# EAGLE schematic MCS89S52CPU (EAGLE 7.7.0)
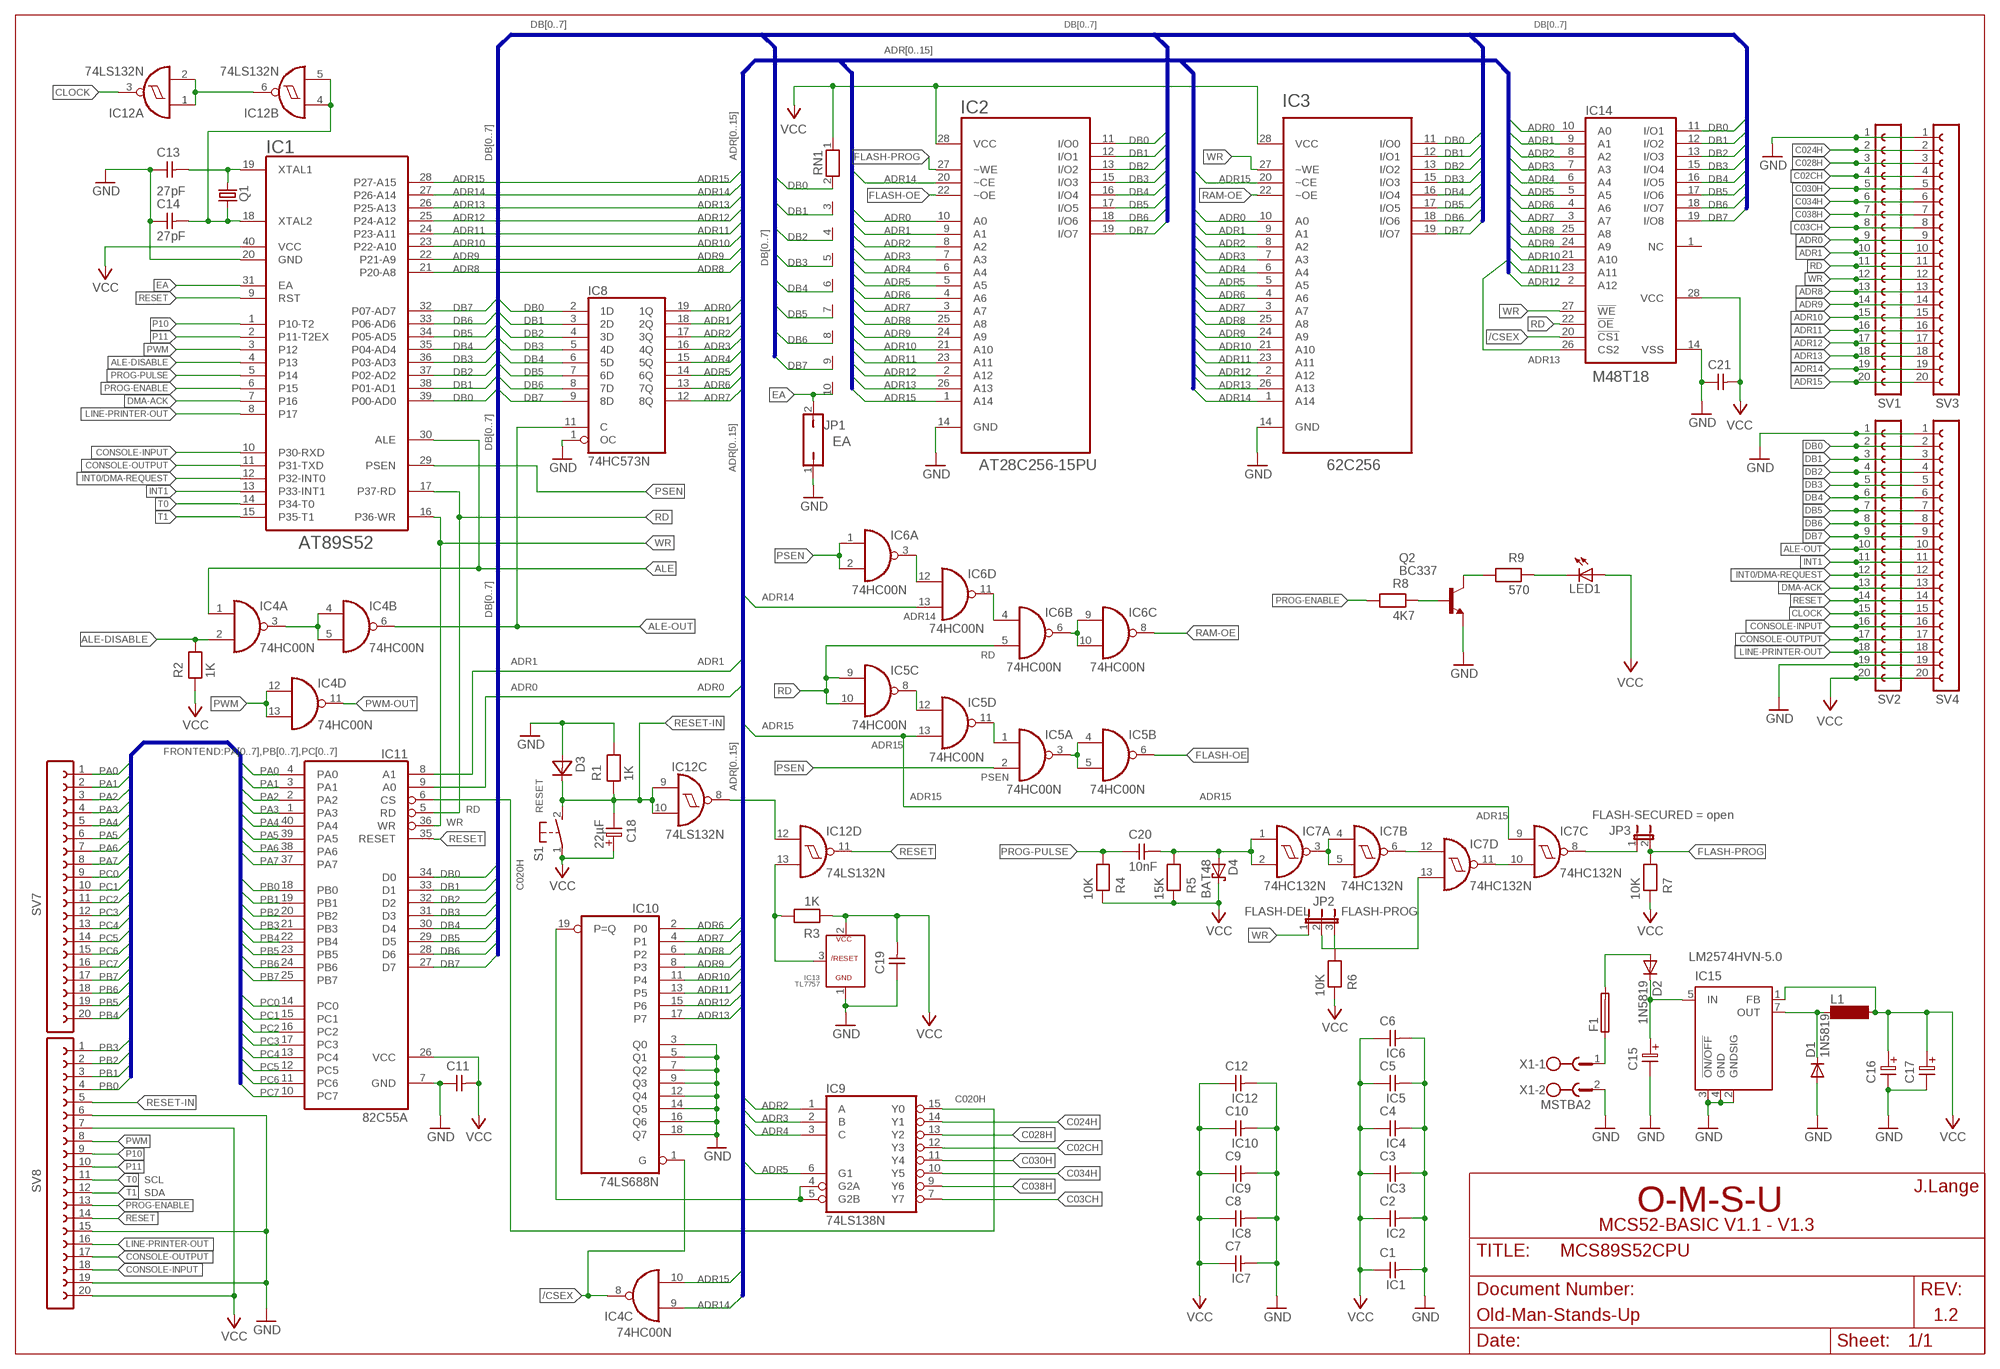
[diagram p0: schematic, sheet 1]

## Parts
C1  CAPNP-5  [C-5]
C2  CAPNP-5  [C-5]
C3  CAPNP-5  [C-5]
C4  CAPNP-5  [C-5]
C5  CAPNP-5  [C-5]
C6  CAPNP-5  [C-5]
C7  CAPNP-5  [C-5]
C8  CAPNP-5  [C-5]
C9  CAPNP-5  [C-5]
C10  CAPNP-5  [C-5]
C11  CAPNP-5  [C-5]
C12  CAPNP-5  [C-5]
C13  27pF  CAPNP-2,5  [C-2,5]
C14  27pF  CAPNP-2,5  [C-2,5]
C15  ELC-5  [ES-5]
C16  ELC-5  [ES-5]
C17  ELC-5  [ES-5]
C18  22µF  ELC-2,5  [ES-2,5]
C19  CAPNP-5  [C-5]
C20  10nF  CAPNP-5  [C-5]
C21  CAPNP-5  [C-5]
D1  1N5819  DIODE-DO41-7.6  [DO41-7.6]
D2  1N5819  DIODE-DO41-7.6  [DO41-7.6]
D3  DIODE-7,5  [D-7,5]
D4  BAT48  BAT42  [DO35-10]
F1  TR5  [TR5]
IC1  AT89S52  8052N  [DIL40]
IC2  AT28C256-15PU  [DIP254P1524X482-28]
IC3  62C256  AT28C256-15PU  [DIP254P1524X482-28]
IC4  74HC00N  [DIL14]
IC5  74HC00N  [DIL14]
IC6  74HC00N  [DIL14]
IC7  74HC132N  [DIL14]
IC8  74HC573N  [DIL20]
IC9  74LS138N  [DIL16]
IC10  74LS688N  [DIL20]
IC11  82C55A  [DIL40]
IC12  74LS132N  [DIL14]
IC13  TL7757  [TO92]
IC14  M48T18  6264A  [DIL28-6]
IC15  LM2574HVN-5.0  [DIL08]
JP1  JP1Q  [JP1]
JP2  JP2E  [JP2]
JP3  JP1E  [JP1]
L1  12K100-7,5  [12K100-7.5]
LED1  LED5MM  [LED5MM]
Q1  CRYSTALHC49S  [HC49/S]
Q2  BC337  [TO92]
R1  1K  RESEU-7,5  [R-7,5]
R2  1K  RESEU-7,5  [R-7,5]
R3  1K  RESEU-7,5  [R-7,5]
R4  10K  RESEU-7,5  [R-7,5]
R5  15K  RESEU-7,5  [R-7,5]
R6  10K  RESEU-7,5  [R-7,5]
R7  10K  RESEU-7,5  [R-7,5]
R8  4K7  RESEU-7,5  [R-7,5]
R9  570  RESEU-7,5  [R-7,5]
RN1  RN09  [RN-10]
S1  31-XX  [B3F-31XX]
SV1  FE20W  [FE20W]
SV2  FE20W  [FE20W]
SV3  FE20-1  [FE20]
SV4  FE20-1  [FE20]
SV7  FE20-1  [FE20]
SV8  FE20-1  [FE20]
X1  MSTBA2  [MSTBA2]

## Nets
/CSEX: IC4.8(C:O) IC10.1(G) IC14.20(!CS1)
ADR0: IC2.10(A0) IC3.10(A0) IC8.19(1Q) IC11.9(A0) IC14.10(A0) SV1.9 SV3.9
ADR1: IC2.9(A1) IC3.9(A1) IC8.18(2Q) IC11.8(A1) IC14.9(A1) SV1.10 SV3.10
ADR2: IC2.8(A2) IC3.8(A2) IC8.17(3Q) IC9.1(A) IC14.8(A2)
ADR3: IC2.7(A3) IC3.7(A3) IC8.16(4Q) IC9.2(B) IC14.7(A3)
ADR4: IC2.6(A4) IC3.6(A4) IC8.15(5Q) IC9.3(C) IC14.6(A4)
ADR5: IC2.5(A5) IC3.5(A5) IC8.14(6Q) IC9.6(G1) IC14.5(A5)
ADR6: IC2.4(A6) IC3.4(A6) IC8.13(7Q) IC10.2(P0) IC14.4(A6)
ADR7: IC2.3(A7) IC3.3(A7) IC8.12(8Q) IC10.4(P1) IC14.3(A7)
ADR8: IC1.21(P20-A8) IC2.25(A8) IC3.25(A8) IC10.6(P2) IC14.25(A8) SV1.13 SV3.13
ADR9: IC1.22(P21-A9) IC2.24(A9) IC3.24(A9) IC10.8(P3) IC14.24(A9) SV1.14 SV3.14
ADR10: IC1.23(P22-A10) IC2.21(A10) IC3.21(A10) IC10.11(P4) IC14.21(A10) SV1.15 SV3.15
ADR11: IC1.24(P23-A11) IC2.23(A11) IC3.23(A11) IC10.13(P5) IC14.23(A11) SV1.16 SV3.16
ADR12: IC1.25(P24-A12) IC2.2(A12) IC3.2(A12) IC10.15(P6) IC14.2(A12) SV1.17 SV3.17
ADR13: IC1.26(P25-A13) IC2.26(A13) IC3.26(A13) IC10.17(P7) IC14.26(CS2) SV1.18 SV3.18
ADR14: IC1.27(P26-A14) IC2.20(~CE) IC3.1(A14) IC4.9(C:I0) IC6.13(D:I1) SV1.19 SV3.19
ADR15: IC1.28(P27-A15) IC2.1(A14) IC3.20(~CE) IC4.10(C:I1) IC5.13(D:I1) IC7.9(C:I0) SV1.20 SV3.20
ALE: IC1.30(ALE) IC4.1(A:I0)
ALE-DISABLE: IC1.4(P13) IC4.2(A:I1) R2.2
ALE-OUT: IC4.6(B:O) IC8.11(C) SV2.10 SV4.10
C02CH: IC9.12(Y3) SV1.4 SV3.4
C03CH: IC9.7(Y7) SV1.8 SV3.8
C020H: IC9.15(Y0) IC11.6(CS)
C024H: IC9.14(Y1) SV1.2 SV3.2
C028H: IC9.13(Y2) SV1.3 SV3.3
C030H: IC9.11(Y4) SV1.5 SV3.5
C034H: IC9.10(Y5) SV1.6 SV3.6
C038H: IC9.9(Y6) SV1.7 SV3.7
CLOCK: IC12.3(A:O) SV2.15 SV4.15
CONSOLE-INPUT: IC1.10(P30-RXD) SV2.16 SV4.16 SV8.18
CONSOLE-OUTPUT: IC1.11(P31-TXD) SV2.17 SV4.17 SV8.17
DB0: IC1.39(P00-AD0) IC2.11(I/O0) IC3.11(I/O0) IC8.2(1D) IC11.34(D0) IC14.11(I/O1) RN1.2 SV2.2 SV4.2
DB1: IC1.38(P01-AD1) IC2.12(I/O1) IC3.12(I/O1) IC8.3(2D) IC11.33(D1) IC14.12(I/O2) RN1.3 SV2.3 SV4.3
DB2: IC1.37(P02-AD2) IC2.13(I/O2) IC3.13(I/O2) IC8.4(3D) IC11.32(D2) IC14.13(I/O3) RN1.4 SV2.4 SV4.4
DB3: IC1.36(P03-AD3) IC2.15(I/O3) IC3.15(I/O3) IC8.5(4D) IC11.31(D3) IC14.15(I/O4) RN1.5 SV2.5 SV4.5
DB4: IC1.35(P04-AD4) IC2.16(I/O4) IC3.16(I/O4) IC8.6(5D) IC11.30(D4) IC14.16(I/O5) RN1.6 SV2.6 SV4.6
DB5: IC1.34(P05-AD5) IC2.17(I/O5) IC3.17(I/O5) IC8.7(6D) IC11.29(D5) IC14.17(I/O6) RN1.7 SV2.7 SV4.7
DB6: IC1.33(P06-AD6) IC2.18(I/O6) IC3.18(I/O6) IC8.8(7D) IC11.28(D6) IC14.18(I/O7) RN1.8 SV2.8 SV4.8
DB7: IC1.32(P07-AD7) IC2.19(I/O7) IC3.19(I/O7) IC8.9(8D) IC11.27(D7) IC14.19(I/O8) RN1.9 SV2.9 SV4.9
DMA-ACK: IC1.7(P16) SV2.13 SV4.13
EA: IC1.31(EA) JP1.2 RN1.10
FLASH-OE: IC2.22(~OE) IC5.6(B:O)
FLASH-PROG: IC2.27(~WE) JP3.2 R7.1
GND: C1.2 C2.2 C3.2 C4.2 C5.2 C6.2 C7.2 C8.2 C9.2 C10.2 C11.1 C12.2 C13.1 C14.1 C15.2 C16.2 C17.2 C19.1 C21.1 D1.A D3.1(A) IC1.20(GND) IC2.14(GND) IC3.14(GND) IC8.1(OC) IC10.3(Q0) IC10.5(Q1) IC10.7(Q2) IC10.9(Q3) IC10.12(Q4) IC10.14(Q5) IC10.16(Q6) IC10.18(Q7) IC11.7(GND) IC13.1(GND) IC14.14(VSS) IC15.2(GNDSIG) IC15.3(!ON/OFF) IC15.4(GND) JP1.1 Q2.1(E) R1.2 SV1.1 SV2.1 SV2.19 SV3.1 SV4.1 SV4.19 SV8.6 SV8.15 SV8.19 X1.2
INT0/DMA-REQUEST: IC1.12(P32-INT0) SV2.12 SV4.12
INT1: IC1.13(P33-INT1) SV2.11 SV4.11
LINE-PRINTER-OUT: IC1.8(P17) SV2.18 SV4.18 SV8.16
N$1: D1.C IC15.7(OUT) L1.1
N$2: C13.2 IC1.19(XTAL1) Q1.2
N$3: C15.1 D2.C IC15.5(IN)
N$4: F1.1 X1.1
N$5: D2.A F1.2
N$6: C14.2 IC1.18(XTAL2) IC12.4(B:I0) IC12.5(B:I1) Q1.1
N$7: IC12.13(D:I1) IC13.3(/RESET) R3.2
N$8: IC4.3(A:O) IC4.4(B:I0) IC4.5(B:I1)
N$9: IC12.1(A:I0) IC12.2(A:I1) IC12.6(B:O)
N$10: IC5.8(C:O) IC5.12(D:I0)
N$11: IC5.1(A:I0) IC5.11(D:O)
N$12: IC12.8(C:O) IC12.12(D:I0)
N$13: IC5.3(A:O) IC5.4(B:I0) IC5.5(B:I1)
N$14: IC6.3(A:O) IC6.12(D:I0)
N$15: IC6.4(B:I0) IC6.11(D:O)
N$16: IC6.6(B:O) IC6.9(C:I0) IC6.10(C:I1)
N$17: IC7.3(A:O) IC7.4(B:I0) IC7.5(B:I1)
N$18: C20.2 D4.A IC7.1(A:I0) IC7.2(A:I1) R5.1
N$19: IC7.6(B:O) IC7.12(D:I0)
N$20: IC7.10(C:I1) IC7.11(D:O)
N$21: IC7.13(D:I1) JP2.2
N$22: JP2.3 R6.1
N$23: Q2.2(B) R8.2
N$24: IC7.8(C:O) JP3.1
N$25: Q2.3(C) R9.1
N$26: LED1.K(C) R9.2
N$29: IC9.4(G2A) IC9.5(G2B) IC10.19(P=Q)
P10: IC1.1(P10-T2) SV8.9
P11: IC1.2(P11-T2EX) SV8.10
PA0: IC11.4(PA0) SV7.1
PA1: IC11.3(PA1) SV7.2
PA2: IC11.2(PA2) SV7.3
PA3: IC11.1(PA3) SV7.4
PA4: IC11.40(PA4) SV7.5
PA5: IC11.39(PA5) SV7.6
PA6: IC11.38(PA6) SV7.7
PA7: IC11.37(PA7) SV7.8
PB0: IC11.18(PB0) SV8.4
PB1: IC11.19(PB1) SV8.3
PB2: IC11.20(PB2) SV8.2
PB3: IC11.21(PB3) SV8.1
PB4: IC11.22(PB4) SV7.20
PB5: IC11.23(PB5) SV7.19
PB6: IC11.24(PB6) SV7.18
PB7: IC11.25(PB7) SV7.17
PC0: IC11.14(PC0) SV7.9
PC1: IC11.15(PC1) SV7.10
PC2: IC11.16(PC2) SV7.11
PC3: IC11.17(PC3) SV7.12
PC4: IC11.13(PC4) SV7.13
PC5: IC11.12(PC5) SV7.14
PC6: IC11.11(PC6) SV7.15
PC7: IC11.10(PC7) SV7.16
PROG-ENABLE: IC1.6(P15) R8.1 SV8.13
PROG-PULSE: C20.1 IC1.5(P14) R4.1
PSEN: IC1.29(PSEN) IC5.2(A:I1) IC6.1(A:I0) IC6.2(A:I1)
PWM: IC1.3(P12) IC4.12(D:I0) IC4.13(D:I1) SV8.8
PWM-OUT: IC4.11(D:O)
RAM-OE: IC3.22(~OE) IC6.8(C:O)
RD: IC1.17(P37-RD) IC5.9(C:I0) IC5.10(C:I1) IC6.5(B:I1) IC11.5(RD) IC14.22(!OE) SV1.11 SV3.11
RESET: IC1.9(RST) IC11.35(RESET) IC12.11(D:O) SV2.14 SV4.14 SV8.14
RESET-IN: C18.2 D3.2(K) IC12.9(C:I0) IC12.10(C:I1) R1.1 S1.2(S) SV8.5
T0: IC1.14(P34-T0) SV8.11
T1: IC1.15(P35-T1) SV8.12
VCC: C1.1 C2.1 C3.1 C4.1 C5.1 C6.1 C7.1 C8.1 C9.1 C10.1 C11.2 C12.1 C16.1 C17.1 C18.1 C19.2 C21.2 D4.C IC1.40(VCC) IC2.28(VCC) IC3.28(VCC) IC11.26(VCC) IC13.2(VCC) IC14.28(VCC) IC15.1(FB) L1.2 LED1.A R2.1 R3.1 R4.2 R5.2 R6.2 R7.2 RN1.1 S1.1(P) SV2.20 SV4.20 SV8.7 SV8.20
WR: IC1.16(P36-WR) IC3.27(~WE) IC11.36(WR) IC14.27(!WE) JP2.1 SV1.12 SV3.12
Unconnected: IC14.1(NC)

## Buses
DB[0..7]
ADR[0..15]
FRONTEND:PA[0..7],PB[0..7],PC[0..7]

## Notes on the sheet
- EA
- RESET
- FLASH-SECURED = open
- FLASH-DEL | FLASH-PROG
- IC6
- IC12 | IC5
- IC10 | IC4
- SCL
- SDA | IC9 | IC3 | J.Lange
- O-M-S-U
- MCS52-BASIC V1.1 - V1.3
- IC8 | IC2
- IC7
- IC1
- Old-Man-Stands-Up | 1.2

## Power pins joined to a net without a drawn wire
GND: IC4.7(P:GND) IC5.7(P:GND) IC6.7(P:GND) IC7.7(P:GND) IC8.10(GND) IC9.8(GND) IC10.10(GND) IC12.7(P:GND)
VCC: IC4.14(P:VCC) IC5.14(P:VCC) IC6.14(P:VCC) IC7.14(P:VCC) IC8.20(VCC) IC9.16(VCC) IC10.20(VCC) IC12.14(P:VCC)

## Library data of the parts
C1-C12 C19-C21 = discrete:CAPNP-5
C13 C14 = discrete:CAPNP-2,5
C15-C17 = discrete:ELC-5
C18 = discrete:ELC-2,5
D1 D2 = diode:DIODE-: DIODE
D3 = discrete:DIODE-7,5
D4 = diode:BAT42: DIODE
F1 = fuse:TR5: FUSE; OC_FARNELL: unknown; OC_NEWARK: unknown
IC1 = micro-intel:8052: MICROCOMPUTER/PERIPHERAL DEVICE 80C51/87C51/80C52/87C52 80C51 8-bit microcontroller family 4 K/8 K OTP/ROM low voltage (2.7 V-5.5 V), low power, high speed (33 MHz), 128/256 B RAM Source: www.semiconductors.philips.com .. 8XC51_8XC52_6.pdf; OC_FARNELL: unknown; OC_NEWARK: unknown
IC2 IC3 = Atmel_By_element14_Batch_1-00:AT28C256-15PU: Paged Parallel EEPROM; DESCRIPTION: Paged Parallel EEPROM; MPN: AT28C256-15PU; OC_FARNELL: 1095782; OC_NEWARK: 96K6555; PACKAGE: PDIP-28; SUPPLIER: ATMEL
IC4-IC6 = 74xx-eu:74*00: Quad 2-input NAND gate
IC7 IC12 = 74xx-eu:74*132: Quad 2-input NAND schmitt trigger
IC8 = 74xx-eu:74*573: 8-bit D latch BUS DRIVER
IC9 = 74xx-eu:74*138: 3-line to 8-line DECODER/DEMULTIPLEXER
IC10 = 74xx-eu:74*688: 8-bit MAGNITUDE/IDENTITY COMPARATOR, totem pole
IC11 = micro-intel:82C55A: MICROCOMPUTER/PERIPHERAL DEVICE; MF: INTERSIL; MPN: IP82C55AZ; OC_FARNELL: 1562050; OC_NEWARK: 79K6939
IC13 = IC:TL7757
IC14 = memory-hitachi:6264A: MEMORY; OC_FARNELL: 283605; OC_NEWARK: unknown
IC15 = linear:LM2574?-*: SIMPLE SWITCHER 0.5A Step-Down Voltage Regulator Source: http://cache.national.com/ds/LM/LM2574.pdf
JP1 = jumper:JP1Q: JUMPER
JP2 = jumper:JP2E: JUMPER
JP3 = jumper:JP1E: JUMPER
L1 = inductor-neosid:12K100-7,5
LED1 = led:LED: LED
Q1 = crystal:CRYSTAL: CRYSTAL; OC_FARNELL: 1667008; OC_NEWARK: unknown
Q2 = transistor-npn:BC337*: NPN Transistor
R1-R9 = discrete:RESEU-7,5
RN1 = resistor-net:RN09: RESISTOR NETWORK; OC_FARNELL: unknown; OC_NEWARK: unknown
S1 = switch-omron:31-XX: OMRON SWITCH; MPN: B3F-3100; OC_FARNELL: 959704; OC_NEWARK: 36M3582
SV1 SV2 = con-lsta:FE20W: FEMALE HEADER; OC_FARNELL: unknown; OC_NEWARK: unknown
SV3 SV4 SV7 SV8 = con-lsta:FE20-1: FEMALE HEADER; OC_FARNELL: unknown; OC_NEWARK: unknown
X1 = con-phoenix-508:MSTBA2: PHOENIX; MF: FARNELL; MPN: 1757242; OC_FARNELL: 3705171; OC_NEWARK: 71C4161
